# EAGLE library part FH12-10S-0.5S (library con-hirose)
0.5mm Pitch Connectors For FPC/FFC Source: Data sheet
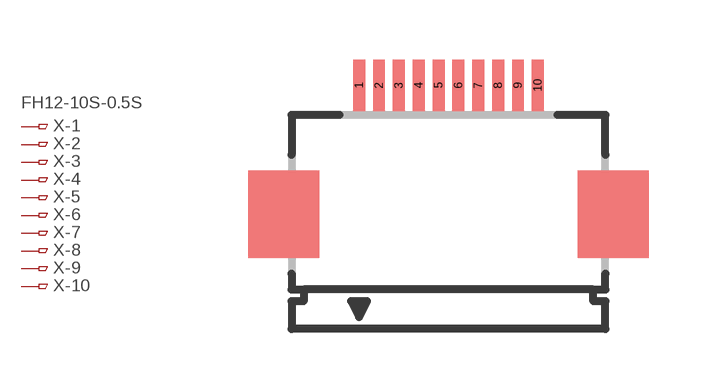
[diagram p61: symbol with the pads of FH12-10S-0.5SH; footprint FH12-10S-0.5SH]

Designator prefix X; gates -1=PINV -2=PIN -3=PIN -4=PIN -5=PIN -6=PIN -7=PIN -8=PIN -9=PIN -10=PIN

## FH12-10S-0.5SH (MPN: FH12-10S-0.5SH(55); OC_FARNELL: 1324540; OC_NEWARK: 34M6152)  [FH12-10S-0.5SH]
1  -1:1  pas
2  -2:1  pas
3  -3:1  pas
4  -4:1  pas
5  -5:1  pas
6  -6:1  pas
7  -7:1  pas
8  -8:1  pas
9  -9:1  pas
10  -10:1  pas

## Footprint FH12-10S-0.5SH (pad centres in mm)
0.5mm Pitch Connectors For FPC/FFC Source: Data sheet
smd 0.3 x 1.3: 1 -2.25,3.25; 2 -1.75,3.25; 3 -1.25,3.25; 4 -0.75,3.25; 5 -0.25,3.25; 6 0.25,3.25; 7 0.75,3.25; 8 1.25,3.25; 9 1.75,3.25; 10 2.25,3.25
